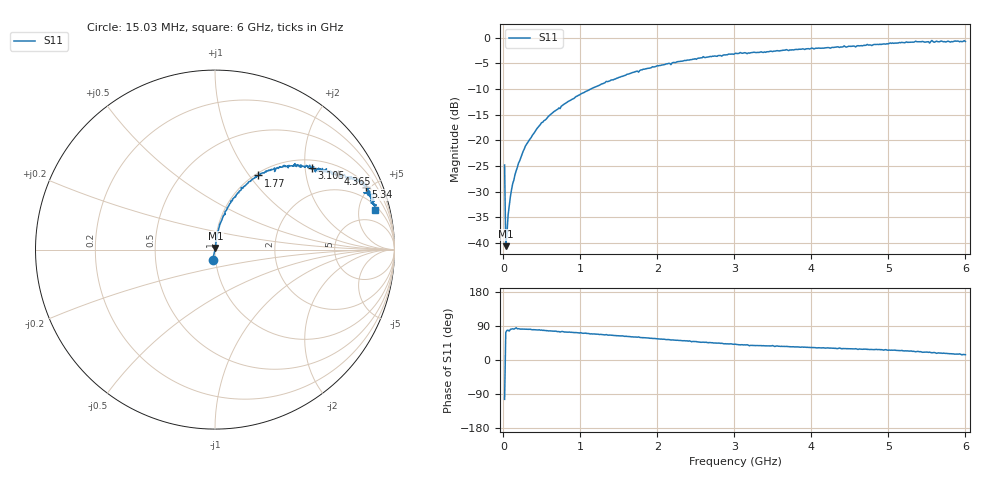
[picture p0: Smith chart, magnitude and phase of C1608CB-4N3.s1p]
!	Network	Analyzer	HP8753E.07.74:	Oct	30	2002	Serial	No.	JP38451487
!	Hewlett-Packard
!	27	Aug	2009	16:19:50
!	Frequency	S11
#	HZ	S	RI	R	50
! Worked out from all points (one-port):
!   400 points, 15.03 MHz to 6 GHz, reference 50 ohm
!   lowest |S11| = -40.6 dB at 30.03 MHz (marker M1), VSWR 1.02, Z = 50.3 + j0.893 ohm
!   |S11| at or under -10 dB: start of sweep to 1.133 GHz
!   S11 on the Smith chart (normalised r, x): 15.03 MHz: 0.97, -0.11; 1.77 GHz: 1.03, +1.11; 3.105 GHz: 1.19, +2.17; 4.365 GHz: 1.28, +3.05; 5.34 GHz: 1.14, +4.75; 6 GHz: 2.50, +7.29
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1.502992e7  -0.0137 -0.0558
3.002985e7  0.00277 0.00888
4.502978e7  0.00251 0.0118
6.00297e7  0.00369 0.0182
1.050295e8  0.00488 0.0327
1.500292e8  0.00572 0.046
2.550287e8  0.0115 0.0771
4.950275e8  0.028 0.146
7.650262e8  0.0555 0.212
1.335023e9  0.146 0.346
1.515022e9  0.184 0.37
1.770021e9  0.242 0.413
2.265019e9  0.359 0.462
3.015015e9  0.528 0.47
3.105014e9  0.539 0.456
3.765011e9  0.623 0.436
4.335008e9  0.708 0.405
4.365008e9  0.685 0.421
4.425008e9  0.721 0.418
4.515007e9  0.718 0.404
5.265004e9  0.828 0.361
5.340003e9  0.842 0.35
5.520002e9  0.86 0.315
5.535002e9  0.829 0.317
5.565002e9  0.889 0.309
5.595002e9  0.85 0.307
5.625002e9  0.884 0.28
6e9  0.893 0.223
